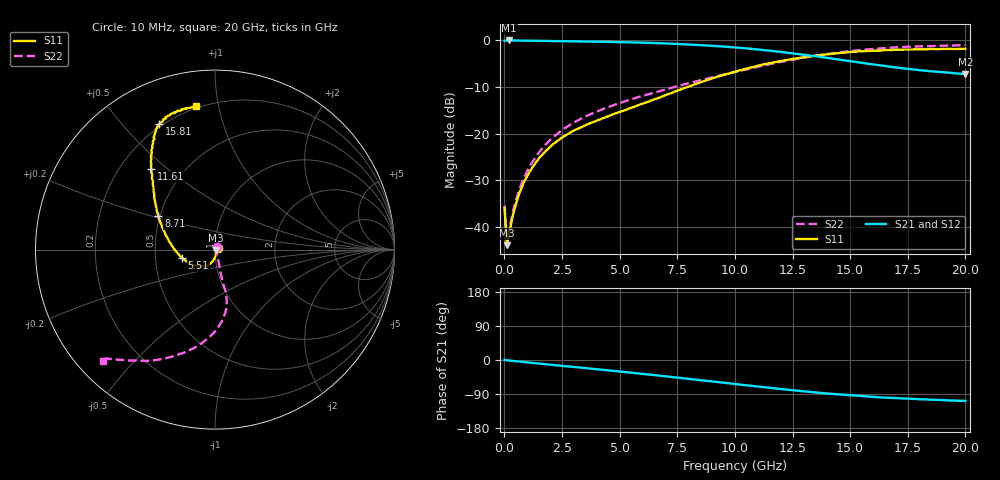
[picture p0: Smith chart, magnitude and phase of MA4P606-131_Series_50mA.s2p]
! AWR Design Environment (9226) Thu Aug 19 15:24:37 2021
! Document = '50mA'
! nPorts: 2, nXvals: 201
# GHz S DB R 50
!Freq DBS11 AngS11 DBS21 AngS21 DBS12 AngS12 DBS22 AngS22
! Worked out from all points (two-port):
!   201 points, 10 MHz to 20 GHz, reference 50 ohm
!   highest |S21| = -0.10 dB at 210 MHz (marker M1); lowest = -7.2 dB at 20 GHz (marker M2)
!   |S21| within 3 dB of the highest: start of sweep to 12.92 GHz
!   lowest |S11| = -43.9 dB at 110 MHz (marker M3), VSWR 1.01, Z = 50.6 - j0.304 ohm
!   |S11| at or under -10 dB: start of sweep to 7.965 GHz
!   |S22| runs from -44.1 to -1.1 dB; largest |S21 - S12| = 0.027
!   S11 on the Smith chart (normalised r, x): 10 MHz: 1.03, +0.02; 5.51 GHz: 0.69, -0.07; 8.71 GHz: 0.49, +0.21; 11.61 GHz: 0.33, +0.44; 15.81 GHz: 0.19, +0.63; 20 GHz: 0.19, +0.86
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0.01  -35.94 27.5  -0.16 0.7  -0.14 0.7  -35.41 56.3
0.11  -43.87 -27.9  -0.10 -0.8  -0.09 -0.7  -44.07 -27.9
0.21  -41.23 -47.1  -0.10 -1.5  -0.09 -1.4  -40.78 -43.3
0.41  -36.64 -65.0  -0.11 -2.7  -0.10 -2.7  -35.97 -59.9
0.61  -33.32 -74.8  -0.12 -4.0  -0.11 -3.9  -32.54 -65.7
0.91  -29.81 -83.7  -0.14 -5.9  -0.13 -5.7  -28.82 -69.4
1.21  -27.27 -90.1  -0.16 -7.7  -0.14 -7.5  -26.11 -71.5
1.61  -24.70 -97.5  -0.19 -10.1  -0.17 -9.9  -23.36 -73.1
2.11  -22.30 -106.0  -0.23 -13.1  -0.21 -12.8  -20.81 -74.7
2.61  -20.50 -114.7  -0.26 -16.1  -0.25 -15.6  -18.87 -75.8
3.41  -18.44 -128.3  -0.32 -20.8  -0.30 -20.2  -16.63 -76.5
5.51  -14.50 -165.6  -0.51 -33.5  -0.50 -32.7  -12.66 -75.9
6.71  -12.33 174.5  -0.68 -41.2  -0.66 -40.3  -10.96 -76.8
8.71  -8.72 149.2  -1.15 -54.5  -1.12 -53.2  -8.36 -82.9
10.01  -6.79 137.6  -1.59 -63.5  -1.53 -61.8  -6.85 -89.9
11.61  -4.86 128.3  -2.34 -74.2  -2.23 -72.5  -5.06 -101.8
13.41  -3.40 121.2  -3.42 -84.9  -3.28 -83.8  -3.43 -115.4
14.51  -2.78 117.4  -4.19 -90.8  -4.03 -89.8  -2.67 -122.7
15.81  -2.34 114.0  -5.09 -96.6  -4.99 -95.8  -2.00 -129.3
16.71  -2.18 111.1  -5.70 -99.9  -5.66 -99.1  -1.66 -132.1
19.01  -1.90 103.5  -6.88 -105.7  -7.03 -105.4  -1.23 -135.3
20  -1.89 97.5  -7.24 -108.3  -7.47 -107.1  -1.11 -135.0
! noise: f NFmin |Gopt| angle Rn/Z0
0.01  0  1  0  2e-20
2.21  0  1  0  2e-20
4.41  0  1  0  2e-20
6.61  0  1  0  2e-20
8.81  0  1  0  2e-20
11.11  0  1  0  2e-20
13.31  0  1  0  2e-20
15.51  0  1  0  2e-20
17.71  0  1  0  2e-20
20  0  1  0  2e-20
